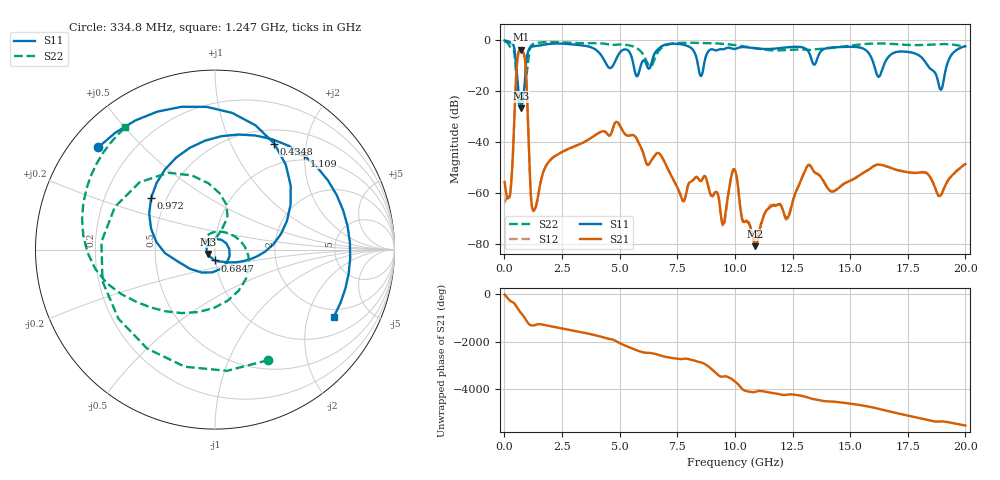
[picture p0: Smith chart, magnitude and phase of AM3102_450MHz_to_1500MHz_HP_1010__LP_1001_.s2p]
!Agilent Technologies,E8364B,MY43040894,A.07.50.67
!Agilent E8364B: A.07.50.67
!Date: Thursday, January 11, 2018 06:12:32
!Correction: S11(Full 2 Port(1,2))
!S21(Full 2 Port(1,2))
!S12(Full 2 Port(1,2))
!S22(Full 2 Port(1,2))
!S2P File: Measurements: S11, S21, S12, S22:
# Hz S  dB  R 50
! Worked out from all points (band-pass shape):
!   1601 points, 10 MHz to 20 GHz, reference 50 ohm
!   highest |S21| = -3.70 dB at 709.6 MHz (marker M1); lowest = -80.7 dB at 10.89 GHz (marker M2)
!   |S21| within 3 dB of the highest: 575.6 MHz to 878.5 MHz (302.9 MHz wide, 41.7 % of centre)
!   lowest |S11| = -26.7 dB at 722.1 MHz (marker M3), VSWR 1.10, Z = 46.1 - j2.22 ohm
!   |S11| at or under -10 dB: 512 MHz to 931.5 MHz (419.4 MHz wide, 58.1 % of centre); 16.05 GHz to 16.45 GHz (401.3 MHz wide, 2.47 % of centre); 18.37 GHz to 19.19 GHz (817.1 MHz wide, 4.35 % of centre)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
!   |S22| runs from -25.6 to -0.4 dB; largest |S21 - S12| = 0.0011
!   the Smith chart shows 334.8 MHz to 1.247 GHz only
!   S11 on the Smith chart (normalised r, x): 334.8 MHz: 0.08, +0.37; 434.8 MHz: 0.68, +1.48; 684.7 MHz: 0.99, -0.12; 972 MHz: 0.41, +0.30; 1.109 GHz: 0.90, +1.98; 1.247 GHz: 1.65, -2.94
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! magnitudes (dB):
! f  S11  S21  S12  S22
! 10 MHz  -0.1  -55.6  -63.4  -0.4
! 334.8 MHz  -1.3  -50.8  -50.9  -3.3
! 434.8 MHz  -3.4  -29.6  -29.5  -5.0
! 684.7 MHz  -24.4  -3.7  -3.7  -25.1
! 709.6 MHz  -26.4  -3.7  -3.7  -24.4
! 722.1 MHz  -26.7  -3.7  -3.7  -23.2
! 972 MHz  -6.8  -18.9  -18.9  -12.5
! 1.109 GHz  -2.8  -53.4  -53.3  -3.4
! 1.247 GHz  -2.4  -66.5  -66.9  -1.5
! 1.909 GHz  -1.4  -47.8  -47.9  -0.7
! 3.346 GHz  -2.0  -40.4  -40.5  -1.1
! 5.757 GHz  -14.1  -38.9  -38.9  -3.2
! 6.682 GHz  -3.3  -44.2  -44.2  -4.4
! 7.744 GHz  -1.7  -63.0  -63.0  -1.0
! 8.718 GHz  -7.0  -53.5  -53.4  -1.1
! 9.493 GHz  -3.5  -72.0  -72.9  -1.4
! 10.01 GHz  -3.4  -51.0  -50.9  -1.9
! 10.89 GHz  -3.1  -80.7  -78.3  -3.2
! 13.34 GHz  -8.0  -50.2  -50.2  -3.7
! 16.68 GHz  -6.3  -49.7  -49.7  -1.3
! 18.94 GHz  -19.4  -60.7  -61.0  -1.5
! 20 GHz  -2.3  -48.5  -48.6  -2.4
